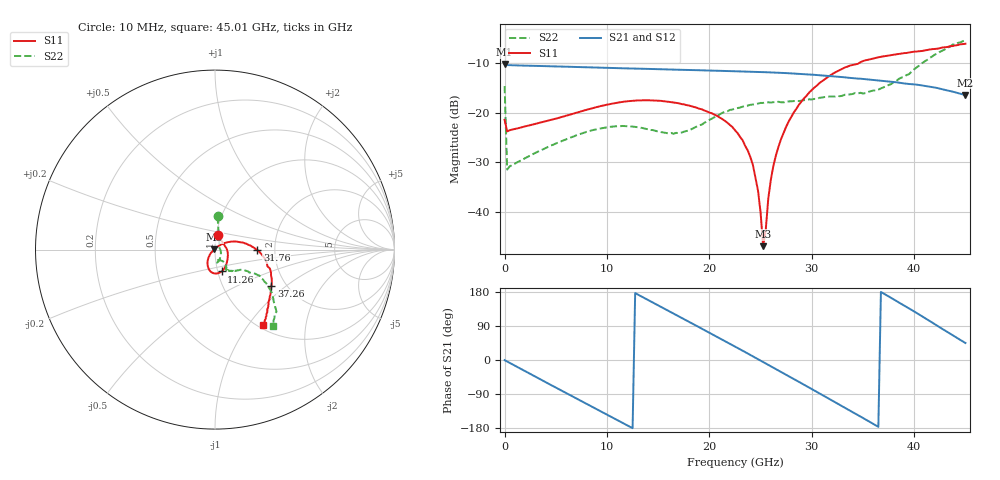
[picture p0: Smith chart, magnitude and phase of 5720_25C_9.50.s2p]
! Device:  ADRF5720
! Description: 0.5dB LSB GaAs MMIC 6-bit Digital Attenuator
! Frequency:  0.000009 -  40 GHz
! Ports:
!	RF1	= Port 1
!	RF2	= Port 2
! Vdd:  3.3 Volt
! Vss:  -3.3 Volt
! Control:  0/3.3 Volt
! State:  9.50 dB attenuation
! Data:  The device was measured using G-S-G Probes on a matrix board.
!  Data was collected using an calibrated 4 port network analyzer.
!  The reference plane for this measurement is at the launchers.
! Note:  Analog Devices supplies this data as a sample of measured data
!  for this product.  Your particular data for this product may vary.
!  Data was taken at 25 degrees C.
!  Analog Devices reserves the right to change this data at anytime.
# GHZ S DB R 45.0
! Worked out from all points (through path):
!   181 points, 10 MHz to 45.01 GHz, reference 45 ohm
!   highest |S21| = -10.21 dB at 10 MHz (marker M1); lowest = -16.4 dB at 45.01 GHz (marker M2)
!   group delay of S21, straight-line fit = 41.3 ps
!   lowest |S11| = -47.0 dB at 25.26 GHz (marker M3), VSWR 1.01, Z = 44.6 + j0.16 ohm
!   |S11| at or under -10 dB: start of sweep to 34.61 GHz
!   |S22| runs from -31.5 to -5.4 dB; largest |S21 - S12| = 0.00042
!   S11 on the Smith chart (normalised r, x): 10 MHz: 1.01, +0.17; 11.26 GHz: 1.04, -0.26; 31.76 GHz: 1.62, -0.01; 37.26 GHz: 1.68, -0.79; 45.01 GHz: 1.06, -1.18
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0.01  -21.43 80.4  -10.21 -0.4  -10.21 -0.4  -14.63 85.6
0.26  -23.79 5.7  -10.39 -4.0  -10.39 -4.0  -31.48 15.2
4.26  -21.61 -31.2  -10.62 -62.0  -10.62 -62.0  -26.90 -45.4
7.76  -19.56 -53.3  -10.82 -112.1  -10.82 -112.1  -24.04 -67.2
11.26  -17.90 -73.3  -11.02 -162.1  -11.02 -162.1  -22.74 -81.4
15.26  -17.61 -93.8  -11.23 140.6  -11.23 140.6  -23.90 -82.8
19.01  -19.20 -109.6  -11.44 86.4  -11.44 86.5  -22.54 -57.8
22.76  -24.12 -127.7  -11.66 31.8  -11.66 31.8  -19.07 -56.2
24.26  -30.58 -140.8  -11.76 9.7  -11.76 9.8  -18.35 -58.8
24.76  -35.76 -147.3  -11.78 2.4  -11.78 2.4  -18.15 -59.5
25.26  -46.95 156.4  -11.82 -5.1  -11.82 -5.1  -18.03 -60.5
25.51  -43.71 71.3  -11.83 -8.8  -11.84 -8.8  -17.93 -61.0
25.76  -37.33 58.8  -11.85 -12.6  -11.86 -12.5  -17.91 -60.8
26.01  -33.53 48.2  -11.87 -16.3  -11.87 -16.2  -17.96 -61.0
26.76  -26.85 40.0  -11.94 -27.6  -11.94 -27.5  -17.80 -60.3
28.26  -19.93 26.1  -12.09 -50.2  -12.10 -50.2  -17.65 -60.5
30.26  -14.93 10.3  -12.36 -80.6  -12.36 -80.6  -17.22 -57.2
31.76  -12.54 -0.7  -12.61 -103.3  -12.61 -103.3  -16.73 -55.2
37.26  -8.55 -32.7  -13.65 171.8  -13.65 171.8  -14.69 -37.7
37.76  -8.37 -34.8  -13.75 164.0  -13.76 164.1  -14.23 -35.3
41.26  -7.36 -46.1  -14.66 107.3  -14.66 107.3  -9.37 -33.2
45.01  -6.08 -57.4  -16.45 44.9  -16.46 45.0  -5.42 -52.7
